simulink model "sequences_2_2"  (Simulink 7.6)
settings: Solver=ode15s  StartTime=0.0  StopTime=10.0  RelTol=1e-3
InitFcn:
  | clear all
  | 
  | clc
  | a=exp(j*2*pi/3);
  | 
  | if exist ('phases_syt_triphase.mat')
  |      load phases_syt_triphase.mat
  | N=length(x);
  | phases=[x(2,N).*exp(j*x(3,N)*pi/180);x(4,N).*exp(j*x(5,N)*pi/180);x(6,N).*exp(j*x(7,N)*pi/180)];
  | 
  | else
  |      clc
  |      error ('le fichier sequence_2_1 soit être exécuté')
  | end
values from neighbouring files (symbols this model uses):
  x = 0:0.001:5    [passe_bande.m]
undefined symbols (not defined in the file or in its folder): j

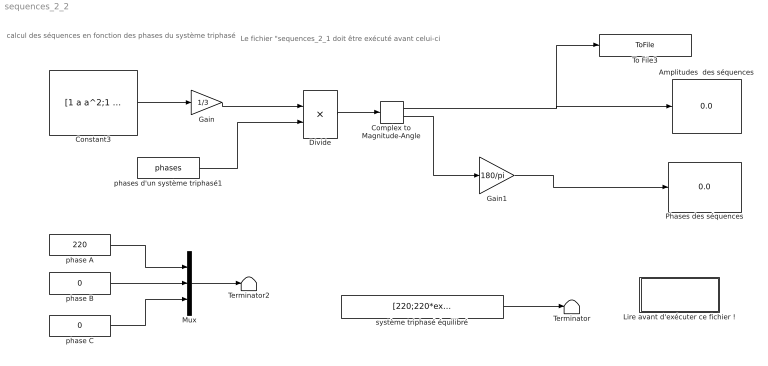
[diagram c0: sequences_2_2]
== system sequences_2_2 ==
  note: calcul des séquences en fonction des phases du système triphasé
  note: Le fichier "sequences_2_1 doit être exécuté avant celui-ci
  Amplitudes  des séquences : Display
  Complex to Magnitude-Angle : ComplexToMagnitudeAngle
  Constant3 : Constant  Value=[1 a a^2;1 a^2 a; 1 1 1]
  Divide : Product  Inputs=**  Multiplication=Matrix(*)
  Gain : Gain  Gain=1/3
  Gain1 : Gain  Gain=180/pi
  Lire avant d'exécuter ce fichier ! : Subsystem  TreatAsAtomicUnit=on
  Mux : Mux  Inputs=3
  Phases des séquences : Display
  Terminator : Terminator
  Terminator2 : Terminator
  To File3 : ToFile  Filename=amplitudes_sequences  MatrixName=x
  phase A : Constant  Value=220
  phase B : Constant  Value=0
  phase C : Constant  Value=0
  phases d'un système triphasé1 : Constant  Value=phases
  système triphasé équilibré : Constant  Value=[220;220*exp(-j*2*pi/3);220*exp(j*2*pi/3)]
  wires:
  Constant3/1 -> Gain/1
  Divide/1 -> Complex to Magnitude-Angle/1
  Complex to Magnitude-Angle/1 -> To File3/1, Amplitudes  des séquences/1
  Gain/1 -> Divide/1
  Gain1/1 -> Phases des séquences/1
  Complex to Magnitude-Angle/2 -> Gain1/1
  phase A/1 -> Mux/1
  phase B/1 -> Mux/2
  phase C/1 -> Mux/3
  système triphasé équilibré/1 -> Terminator/1
  Mux/1 -> Terminator2/1
  phases d'un système triphasé1/1 -> Divide/2

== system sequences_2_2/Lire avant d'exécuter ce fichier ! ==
